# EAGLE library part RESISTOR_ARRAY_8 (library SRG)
Resistor Array, Isolated Example: Bourns 4816P-1-101LF
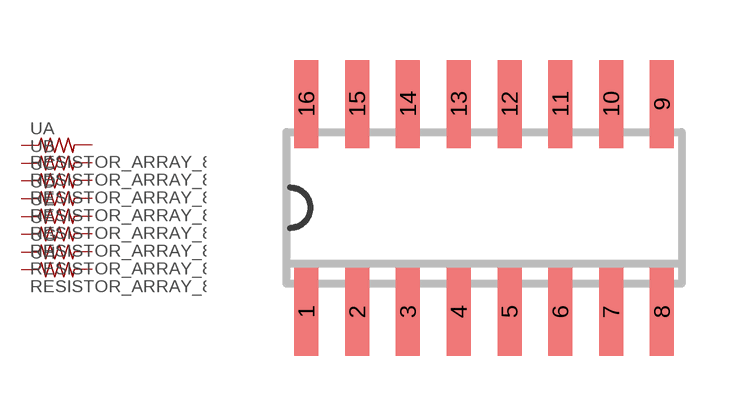
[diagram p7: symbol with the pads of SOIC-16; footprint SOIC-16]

Designator prefix -; gates B=RESISTOR C=RESISTOR D=RESISTOR E=RESISTOR F=RESISTOR G=RESISTOR H=RESISTOR A=RESISTOR

## RESISTOR_ARRAY_8  [SOIC-16]
1  A:1  pas
2  B:1  pas
3  C:1  pas
4  D:1  pas
5  E:1  pas
6  F:1  pas
7  G:1  pas
8  H:1  pas
9  H:2  pas
10  G:2  pas
11  F:2  pas
12  E:2  pas
13  D:2  pas
14  C:2  pas
15  B:2  pas
16  A:2  pas

## Footprint SOIC-16 (pad centres in mm)
SOIC-16
smd 0.6 x 2.2: 1 -4.445,-2.6; 2 -3.175,-2.6; 3 -1.905,-2.6; 4 -0.635,-2.6; 5 0.635,-2.6; 6 1.905,-2.6; 7 3.175,-2.6; 8 4.445,-2.6; 9 4.445,2.6; 10 3.175,2.6; 11 1.905,2.6; 12 0.635,2.6; 13 -0.635,2.6; 14 -1.905,2.6; 15 -3.175,2.6; 16 -4.445,2.6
